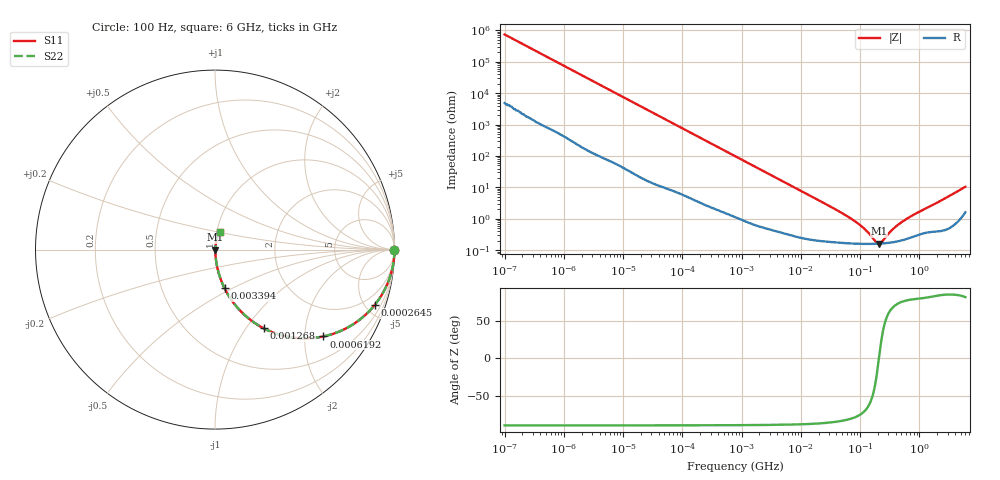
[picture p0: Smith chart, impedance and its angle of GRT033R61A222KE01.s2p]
!Murata Part Number: GRT033R61A222KE01
!These Parameters are Measured in Series Mode Connection
!Data Generated on Jun 19, 2026
!  o--ll--o
!Port1  Port2
!  o------o
!Operation Temp=25[degC], DC Bias Voltage=0[V]
!Freq. Start=100[Hz] Stop=6[GHz] 401[Steps]
# Hz S RI R 50
!Freq.(Hz) S11(Real) S11(Imag) S21(Real) S21(Imag) S12(Real) S12(Imag) S22(Real) S22(Imag)
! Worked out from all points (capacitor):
!   401 points, 100 Hz to 6 GHz, reference 50 ohm
!   read as one part in series: C = 2.14 nF near 109 Hz
!   lowest |Z| = 162 mohm at 208.8 MHz (marker M1)
!   series resonance near 208.4 MHz, so ESL is about 270 pH
!   S11 on the Smith chart (normalised r, x): 100 Hz: open; 264.5 kHz: 1.05, -5.77; 619.2 kHz: 1.03, -2.48; 1.268 MHz: 1.02, -1.22; 3.394 MHz: 1.01, -0.46; 6 GHz: 1.03, +0.21
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100  1 -0.000135  9e-07 0.000135  9e-07 0.000135  1 -0.000135
2008  1 -0.00268  2.08e-05 0.00268  2.08e-05 0.00268  1 -0.00268
40335  0.9968 -0.0531  0.00315 0.0531  0.00315 0.0531  0.9968 -0.0531
112960  0.9773 -0.1451  0.0227 0.1451  0.0227 0.1451  0.9773 -0.1451
264476  0.8906 -0.3077  0.1094 0.3077  0.1094 0.3077  0.8906 -0.3077
395726  0.7865 -0.4049  0.2135 0.4049  0.2135 0.4049  0.7865 -0.4049
619225  0.6043 -0.4836  0.3957 0.4836  0.3957 0.4836  0.6043 -0.4836
774597  0.4959 -0.4943  0.5041 0.4943  0.5041 0.4943  0.4959 -0.4943
1267578  0.2724 -0.4389  0.7276 0.4389  0.7276 0.4389  0.2724 -0.4389
1983483  0.1353 -0.3348  0.8647 0.3348  0.8647 0.3348  0.1353 -0.3348
3394479  0.0532 -0.2153  0.9468 0.2153  0.9468 0.2153  0.0532 -0.2153
6644369  0.0165 -0.1151  0.9835 0.1151  0.9835 0.1151  0.0165 -0.1151
1.555665e7  0.00461 -0.0499  0.9954 0.0499  0.9954 0.0499  0.00461 -0.0499
8.154455e7  0.00168 -0.00825  0.9983 0.00825  0.9983 0.00825  0.00168 -0.00825
1.220122e8  0.0016 -0.00429  0.9984 0.00429  0.9984 0.00429  0.0016 -0.00429
1.825626e8  0.0016 -0.00101  0.9984 0.00101  0.9984 0.00101  0.0016 -0.00101
2.088084e8  0.00162 1.66e-05  0.9984 -1.66e-05  0.9984 -1.66e-05  0.00162 1.66e-05
2.388273e8  0.00164 0.00104  0.9984 -0.00104  0.9984 -0.00104  0.00164 0.00104
3.124326e8  0.00174 0.00317  0.9983 -0.00317  0.9983 -0.00317  0.00174 0.00317
4.274388e8  0.00194 0.00591  0.9981 -0.00591  0.9981 -0.00591  0.00194 0.00591
6.688484e8  0.00252 0.0107  0.9975 -0.0107  0.9975 -0.0107  0.00252 0.0107
6e9  0.026 0.0994  0.974 -0.0994  0.974 -0.0994  0.026 0.0994
